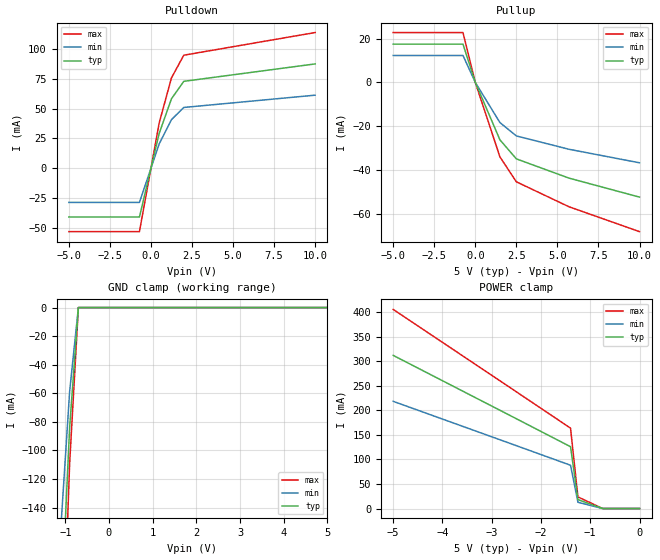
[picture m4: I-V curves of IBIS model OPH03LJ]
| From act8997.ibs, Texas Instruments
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[Model]   OPH03LJ
| 10-mA 3-state CMOS/TTL output buffer with 0.125 di/dt and active-low enable
| OP (97318 ALEY)
| BP (97318 ALEY)
Model_type   3-state
Polarity   Non-Inverting
| Signals   DTDO1-4, TDO
| variable   typ   min   max
C_comp   10pF   NA   NA
| variable   typ   min   max
[Voltage range]   5.0V   4.5V   5.5V
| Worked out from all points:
|   slope of the pulldown table from 0 to 0.75 V, typ, clamps not added: 19.3 ohm
|   slope of the pullup table from 0 to 0.75 V, typ, clamps not added: 57 ohm
|   GND clamp passes 1 mA (typ) near -0.70 V on its own axis
[pullup]
|   50C:5V:   100C:4.5V:weak  0C:5.5V:strong
| Voltage   I(typ)   I(min)   I(max)
-5V       17.5mA     12.3mA     22.8mA
-2.75V    17.5mA     12.3mA     22.8mA
-1.4V     17.5mA     12.3mA     22.8mA
-1.25V    17.5mA     12.3mA     22.8mA
-750mV    17.5mA     12.3mA     22.8mA
0V        0A         0A         0A
1.5V      -26.3mA    -18.4mA    -34.1mA
2.5V      -35mA      -24.5mA    -45.5mA
5.7V      -43.8mA    -30.6mA    -56.9mA
10V       -52.5mA    -36.8mA    -68.3mA
[pulldown]
|   50C:5V:   100C:4.5V:weak  0C:5.5V:strong
| Voltage   I(typ)   I(min)   I(max)
-5V       -40.8mA    -28.6mA    -53.1mA
-900mV    -40.8mA    -28.6mA    -53.1mA
-700mV    -40.8mA    -28.6mA    -53.1mA
-500mV    -29.2mA    -20.4mA    -37.9mA
0V        0A         0A         0A
500mV     29.2mA     20.4mA     37.9mA
1.25V     58.3mA     40.8mA     75.8mA
2V        72.9mA     51mA       94.8mA
10V       87.5mA     61.3mA     113.8mA
[power_clamp]
|   50C:5V:   100C:4.5V:weak  0C:5.5V:strong
| Voltage   I(typ)   I(min)   I(max)
-5V       312.2mA    218.5mA    405.9mA
-2.75V    196mA      137.2mA    254.8mA
-1.4V     126mA      88.2mA     163.8mA
-1.25V    18.2mA     12.7mA     23.7mA
-750mV    0A         0A         0A
0V        0A         0A         0A
[gnd_clamp]
|   50C:5V:   100C:4.5V:weak  0C:5.5V:strong
| Voltage   I(typ)   I(min)   I(max)
-5V       -2.8A      -2A        -3.6A
-900mV    -84mA      -58.8mA    -109.2mA
-700mV    0A         0A         0A
0V        0A         0A         0A
5V        0A         0A         0A
[ramp]
| variable   typ   min   max
dV/dt_r   1.2/2.25e-9   0.9/3.375e-9   1.5/1.5e-9
dV/dt_f   1.8/2e-9   1.5/3e-9   2.1/1.33e-9
